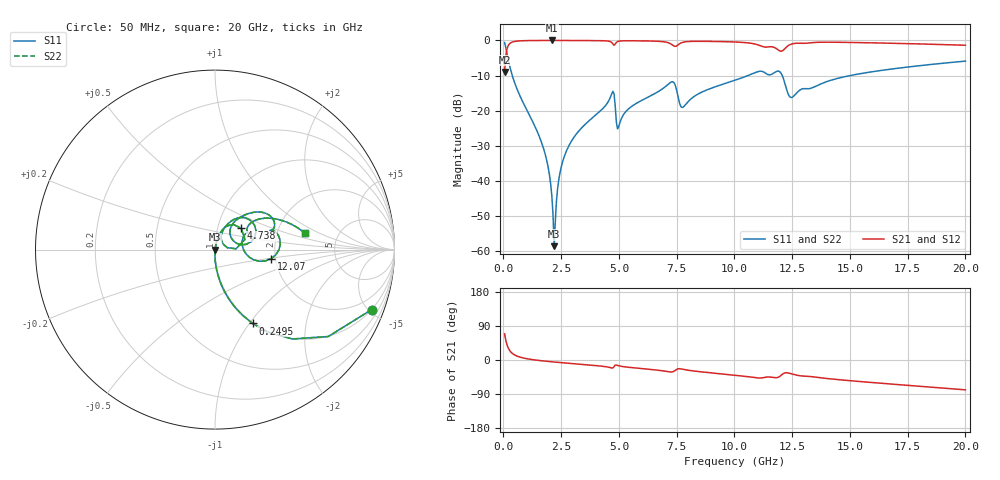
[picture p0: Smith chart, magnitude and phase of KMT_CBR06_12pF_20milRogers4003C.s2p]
! Data measured by Modelithics Inc. support@modelithics.com 813-866-6335
! KEMET CBR0603 12pF, Pad Width= 0.851mm, Pad Length= 0.64mm, Pad Gap= 0.62mm, 20mil Rogers 4003C substrate Data, January 2022
# hz S ma R 50
! 2 Port Network Data from SP1.SP block
! freq  magS11  angS11  magS21  angS21  magS12  angS12  magS22  angS22
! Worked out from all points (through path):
!   401 points, 50 MHz to 20 GHz, reference 50 ohm
!   highest |S21| = -0.01 dB at 2.095 GHz (marker M1); lowest = -9.0 dB at 50 MHz (marker M2)
!   group delay of S21, straight-line fit = 11.6 ps
!   lowest |S11| = -58.5 dB at 2.195 GHz (marker M3), VSWR 1.00, Z = 50.1 - j0.0489 ohm
!   |S11| at or under -10 dB: 383.1 MHz to 10.58 GHz (10.2 GHz wide, 186 % of centre); 12.07 GHz to 15 GHz (2.929 GHz wide, 21.6 % of centre)
!   |S22| runs from -58.5 to -0.6 dB; largest |S21 - S12| = 0
!   S11 on the Smith chart (normalised r, x): 50 MHz: 0.99, -5.23; 249.5 MHz: 0.99, -1.04; 4.738 GHz: 1.30, +0.32; 12.07 GHz: 1.90, -0.21; 20 GHz: 2.86, +0.72
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5e7  0.9346 -20.9  0.3555 69.0  0.3555 69.0  0.9346 -20.9
2.495e8  0.4615 -63.1  0.8866 26.9  0.8866 26.9  0.4615 -63.1
5.98625e8  0.1996 -79.8  0.9792 10.1  0.9792 10.1  0.1996 -79.8
1.74575e9  0.02837 -90.6  0.9985 -2.6  0.9985 -2.6  0.02837 -90.6
1.995125e9  0.01206 -89.1  0.9988 -4.2  0.9988 -4.2  0.01206 -89.1
2.094875e9  0.006165 -84.5  0.9988 -4.8  0.9988 -4.8  0.006165 -84.5
2.194625e9  0.001189 -24.2  0.9988 -5.3  0.9988 -5.3  0.001189 -24.2
2.593625e9  0.02043 79.1  0.9985 -7.5  0.9985 -7.5  0.02043 79.1
3.391625e9  0.05742 76.9  0.9967 -11.5  0.9967 -11.5  0.05742 76.9
4.73825e9  0.1889 39.3  0.8924 -20.9  0.8924 -20.9  0.1889 39.3
4.987625e9  0.05926 50.1  0.9736 -15.2  0.9736 -15.2  0.05926 50.1
5.486375e9  0.1113 67.7  0.9886 -19.7  0.9886 -19.7  0.1113 67.7
6.73325e9  0.19 59.3  0.9701 -27.3  0.9701 -27.3  0.19 59.3
7.33175e9  0.2587 31.5  0.8539 -31.0  0.8539 -31.0  0.2587 31.5
7.780625e9  0.1128 38.1  0.9429 -24.6  0.9429 -24.6  0.1128 38.1
1.0025e10  0.2715 47.4  0.9498 -40.0  0.9498 -40.0  0.2715 47.4
1.097262e10  0.3563 32.9  0.874 -47.1  0.874 -47.1  0.3563 32.9
1.206988e10  0.3174 -9.2  0.7096 -37.9  0.7096 -37.9  0.3174 -9.2
1.246888e10  0.1542 10.1  0.8874 -36.5  0.8874 -36.5  0.1542 10.1
1.336662e10  0.2118 32.8  0.9303 -44.2  0.9303 -44.2  0.2118 32.8
1.670825e10  0.3884 25.7  0.9129 -63.1  0.9129 -63.1  0.3884 25.7
2e10  0.5081 10.5  0.854 -78.7  0.854 -78.7  0.5081 10.5
